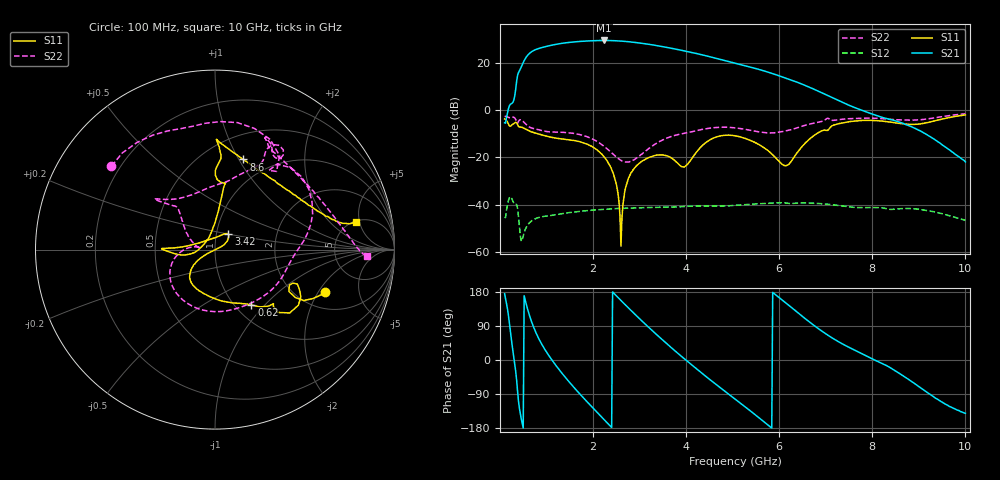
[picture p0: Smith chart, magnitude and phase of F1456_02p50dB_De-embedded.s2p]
! Integrated Device Technology
! Corporate Headquarters
! 6024 Silver Creek Valley Road
! San Jose, CA 95138  USA
! Phone:  1-408-284-8200
! Toll Free:  1-800-223-1366
! Webpage:  http://www.idt.com/
! Timing and RF Division
! 515 Groton Road, Suite 102
! Westford, MA 01886-6024
! Device:  F1456
! Description: 6-bit 0.5 dB Transmit Variable Gain Amplifier
! Frequency:  2100.0 -  2950.00 MHz
! Package:  6x6 mm Thin QFN Plastic Package: 28 pin
! State:  5
! Atten State:  2.5 dB
! Voltage:  +5.00 Volts
! Current:  214.056 mA
! Data:  The device was measured on a the F1455 evaluation board which has
!  individual transmission lines to the RF pins.  Data was collected
!  using a calibrated network analyzer.  The evaluation board was
!  de-embedded using a TRL calibration technique.
!  The reference plane is the edge of the package pin.
!  Pin  1 = CSb
!  Pin  2 = DATA
!  Pin  3 = CLK
!  Pin  4 = RSET
!  Pin  5 = GND
!  Pin  6 = RFIN  = Port 1
!  Pin  7 = GND
!  Pin  8 = NC
!  Pin  9 = NC
!  Pin 10 = NC
!  Pin 11 = NC
!  Pin 12 = NC
!  Pin 13 = NC
!  Pin 14 = /STBY
!  Pin 15 = GND
!  Pin 16 = RFOUT  = Port 2
!  Pin 17 = GND
!  Pin 18 = NC
!  Pin 19 = NC
!  Pin 20 = NC
!  Pin 21 = GND
!  Pin 22 = NC
!  Pin 23 = GND
!  Pin 24 = NC
!  Pin 25 = NC
!  Pin 26 = NC
!  Pin 27 = GND
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# GHz S dB R 50
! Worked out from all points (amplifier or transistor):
!   496 points, 100 MHz to 10 GHz, reference 50 ohm
!   highest |S21| = 29.7 dB at 2.24 GHz (marker M1)
!   |S21| within 3 dB of that: 904.3 MHz to 3.601 GHz (2.696 GHz wide, 120 % of centre)
!   unconditionally stable (mu >= 1): start of sweep to end of sweep
!   at 1.74 GHz: K = 2.22, MAG = 29.9 dB, |S12| = -42.9 dB
!   at 5.06 GHz: K = 4.06, MAG = 21.2 dB, |S12| = -40.4 dB
!   at 10 GHz: K = 139.34, MAG = -12.1 dB, |S12| = -46.7 dB
!   S11 on the Smith chart (normalised r, x): 100 MHz: 2.76, -2.30; 620 MHz: 1.18, -0.84; 3.42 GHz: 1.14, +0.20; 8.6 GHz: 0.75, +1.04; 10 GHz: 5.10, +4.38
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0.1  -3.65 -21.1  -5.26 175.1  -45.38 41.8  -2.61 141.1
0.34  -5.06 -33.8  9.27 -31.2  -39.94 -144.2  -3.94 55.5
0.42  -7.05 -42.7  16.85 -129.1  -49.77 142.5  -4.12 47.2
0.52  -7.64 -50.1  21.15 169.6  -51.94 -166.6  -5.13 15.2
0.62  -8.66 -56.7  23.96 123.2  -48.06 168.3  -6.96 -2.4
0.82  -9.99 -70.0  26.22 59.8  -45.60 118.4  -8.16 -32.2
1.14  -11.57 -95.8  27.82 -4.0  -44.53 72.9  -9.19 -79.3
1.48  -12.49 -118.2  28.87 -56.8  -43.46 44.1  -9.53 -121.0
1.76  -13.58 -132.4  29.36 -95.5  -42.82 25.2  -10.50 -146.6
2.24  -19.79 -148.8  29.72 -157.7  -42.03 -2.6  -15.33 -179.9
2.52  -33.39 -151.7  29.55 167.0  -41.72 -17.6  -20.12 171.4
2.86  -25.28 28.2  28.97 125.4  -41.47 -34.7  -21.18 173.5
3.4  -18.99 48.6  27.43 63.1  -41.19 -60.4  -13.58 144.1
3.42  -18.93 49.2  27.37 60.9  -41.19 -61.5  -13.32 143.3
3.82  -22.53 77.0  25.86 17.9  -41.02 -78.8  -10.31 132.4
4.32  -15.50 173.9  23.72 -33.0  -40.64 -101.8  -8.18 137.7
5.06  -10.81 -179.9  20.05 -103.9  -40.36 -133.1  -7.45 138.3
5.68  -15.94 -169.8  16.73 -163.8  -39.58 -165.2  -9.43 119.2
6.7  -11.39 83.6  9.40 95.6  -39.41 131.6  -5.62 63.2
8.36  -4.90 82.9  -3.70 -18.3  -42.02 59.0  -3.80 62.4
8.6  -5.58 72.5  -5.14 -37.0  -41.79 53.5  -4.04 55.7
10  -1.95 11.2  -21.90 -140.6  -46.68 -22.9  -1.46 -2.5
